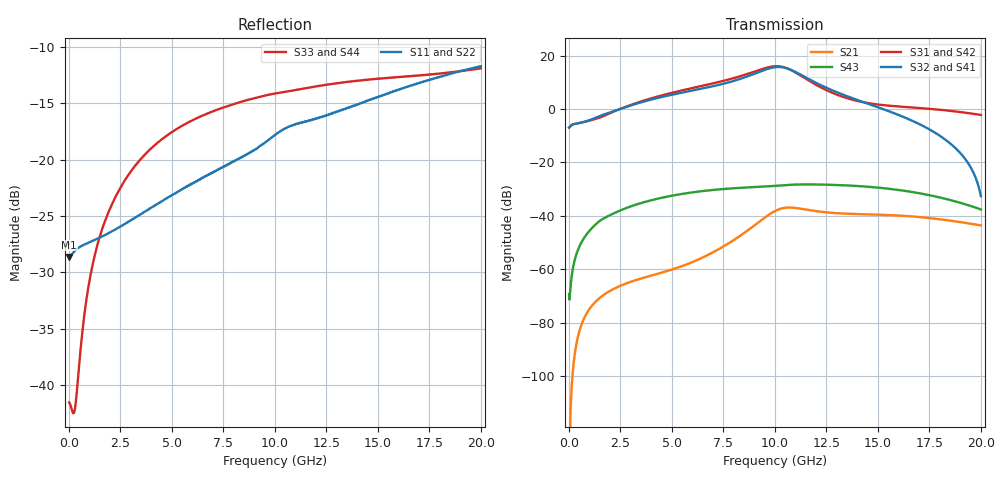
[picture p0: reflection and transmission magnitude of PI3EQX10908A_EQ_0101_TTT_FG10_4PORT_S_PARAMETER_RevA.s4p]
! NPort=4 DATA=2000 NOISE=0 GROUPDELAY=0 COMPLEX_DATAFORMAT=POLAR
! NumOfBlock=1 NumOfParam=0
! .MODEL Smodel S TSTONEFILE=PI3EQX10908A_EQ_0101_TTT_FG10_4PORT_S_PARAMETER_RevA.s4p TYPE=S
!  -- The above .MODEL line can be used for the S element in the netlist.
! The s parameter is extracted from the linear redriver, it is not bi-directional; only s(4,1)s(4,2) and s(3,1)s(3,2)
! should be the insertion loss
!Port definition:
!Port1 = input+
!Port2 = input-
!Port3 = output+
!Port4 = output-
# Hz S MA R  50
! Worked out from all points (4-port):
!   2000 points, 10 MHz to 20 GHz, reference 50 ohm
!   strongest paths, dB at 10 MHz, 5.01 GHz, 10.01 GHz, 15.01 GHz, 20 GHz:
!     S32: -6.9, 5.4, 15.7, 0.6, -32.6
!     S41: -6.9, 5.4, 15.7, 0.6, -32.5
!     S31: -6.9, 6.1, 16.0, 1.7, -2.2
!     S42: -6.9, 6.1, 16.0, 1.7, -2.2
!     S43: -69.4, -32.4, -28.8, -29.4, -37.6
!     S21: -127.2, -60.1, -38.2, -39.6, -43.6
!   lowest |S11| = -28.6 dB at 10 MHz (marker M1), VSWR 1.08, Z = 46.4 - j0.024 ohm
!   |S11| at or under -10 dB: start of sweep to end of sweep
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1e7  0.03701 -179.6  4.342e-07 14.4  0 0.0  0 0.0
     4.342e-07 14.4  0.03701 -179.6  0 0.0  0 0.0
     0.451 1.0  0.451 -179.0  0.008374 26.0  0.00034 -27.1
     0.451 -179.0  0.451 1.0  0.00034 -27.1  0.008374 26.0
7.61e9  0.09388 -117.6  0.002828 132.9  8.619e-07 53.6  3.772e-07 132.3
        0.002827 133.0  0.09391 -117.6  3.772e-07 132.3  8.62e-07 53.6
        3.454 -56.7  3.047 116.6  0.1716 4.6  0.03202 7.0
        3.048 116.7  3.454 -56.7  0.03202 7.0  0.1716 4.6
9.56e9  0.1197 -110.9  0.009579 114.6  3.718e-06 10.5  2.312e-06 119.1
        0.009582 114.6  0.1197 -110.9  2.313e-06 119.1  3.718e-06 10.5
        5.886 -111.7  5.504 62.9  0.1927 -9.9  0.03547 -12.2
        5.505 62.9  5.886 -111.7  0.03547 -12.2  0.1927 -9.9
1.052e10  0.1377 -111.6  0.01417 76.5  5.144e-06 -23.6  5.572e-06 82.4
          0.01417 76.5  0.1378 -111.6  5.574e-06 82.4  5.145e-06 -23.7
          5.921 -161.7  5.871 11.4  0.1999 -16.0  0.03775 -22.0
          5.871 11.4  5.921 -161.7  0.03775 -22.0  0.1999 -16.0
1.151e10  0.148 -113.0  0.01309 44.5  5.278e-06 -32.1  8.468e-06 44.9
          0.01309 44.5  0.148 -113.0  8.471e-06 44.9  5.278e-06 -32.1
          3.663 159.4  3.883 -31.7  0.2074 -21.7  0.03875 -34.6
          3.883 -31.7  3.662 159.4  0.03875 -34.6  0.2074 -21.7
1.365e10  0.171 -111.5  0.01089 15.5  1.384e-05 -38.0  1.707e-05 -4.4
          0.01089 15.6  0.1711 -111.5  1.707e-05 -4.4  1.384e-05 -38.1
          1.534 133.2  1.655 -78.2  0.2217 -32.6  0.03683 -60.6
          1.655 -78.2  1.534 133.2  0.03683 -60.6  0.2217 -32.6
2e10  0.2596 -114.3  0.006632 -42.6  9.078e-05 -147.7  7.233e-05 -137.5
      0.006626 -42.4  0.2597 -114.3  7.233e-05 -137.5  9.076e-05 -147.7
      0.7746 58.9  0.02336 179.3  0.2539 -52.2  0.01316 -136.8
      0.02374 -179.5  0.7752 58.9  0.01316 -136.8  0.2539 -52.2
